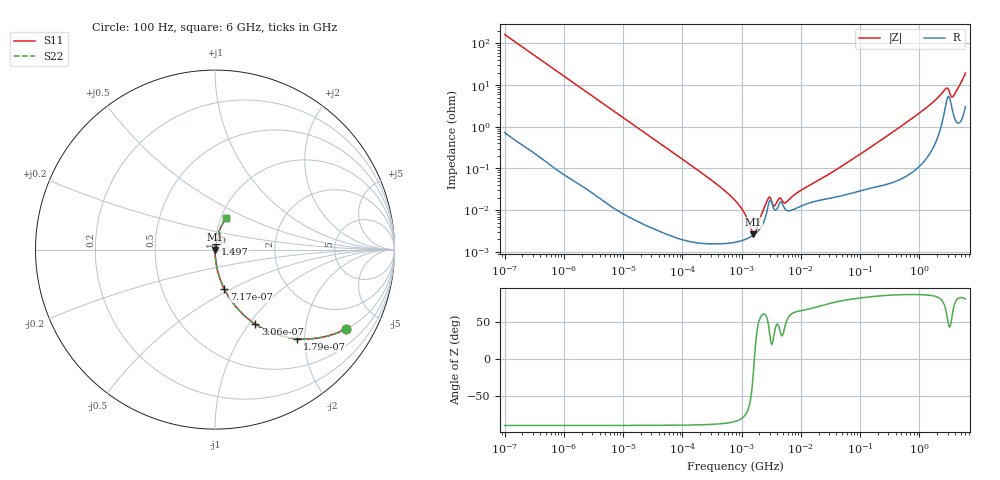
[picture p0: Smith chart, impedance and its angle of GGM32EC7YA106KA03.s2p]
!Murata Part Number: GGM32EC7YA106KA03
!These Parameters are Measured in Series Mode Connection
!Data Generated on Jun 19, 2026
!  o--ll--o
!Port1  Port2
!  o------o
!Operation Temp=25[degC], DC Bias Voltage=0[V]
!Freq. Start=100[Hz] Stop=6[GHz] 401[Steps]
# Hz S RI R 50
!Freq.(Hz) S11(Real) S11(Imag) S21(Real) S21(Imag) S12(Real) S12(Imag) S22(Real) S22(Imag)
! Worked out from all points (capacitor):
!   401 points, 100 Hz to 6 GHz, reference 50 ohm
!   read as one part in series: C = 9.68 uF near 109 Hz
!   lowest |Z| = 2.63 mohm at 1.586 MHz (marker M1)
!   series resonance near 1.645 MHz, so ESL is about 970 pH
!   S11 on the Smith chart (normalised r, x): 100 Hz: 1.01, -3.29; 179 Hz: 1.01, -1.84; 306 Hz: 1.00, -1.08; 717 Hz: 1.00, -0.46; 1.497 GHz: 1.00, +0.07; 6 GHz: 1.06, +0.38
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100  0.7288 -0.4424  0.2712 0.4424  0.2712 0.4424  0.7288 -0.4424
179  0.4582 -0.4961  0.5418 0.4961  0.5418 0.4961  0.4582 -0.4961
306  0.2255 -0.4157  0.7745 0.4157  0.7745 0.4157  0.2255 -0.4157
717  0.0512 -0.2183  0.9488 0.2183  0.9488 0.2183  0.0512 -0.2183
2008  0.00713 -0.0818  0.9929 0.0818  0.9929 0.0818  0.00713 -0.0818
40335  4.83e-05 -0.00414  1 0.00414  1 0.00414  4.83e-05 -0.00414
330837  1.57e-05 -0.000487  1 0.000487  1 0.000487  1.57e-05 -0.000487
774597  1.69e-05 -0.00017  1 0.00017  1 0.00017  1.69e-05 -0.00017
1059725  1.89e-05 -9.48e-05  1 9.48e-05  1 9.48e-05  1.89e-05 -9.48e-05
1585629  2.51e-05 -8e-06  1 8e-06  1 8e-06  2.51e-05 -8e-06
2268635  4.53e-05 7.99e-05  1 -7.99e-05  1 -7.99e-05  4.53e-05 7.99e-05
2837864  0.000133 0.000142  0.9999 -0.000142  0.9999 -0.000142  0.000133 0.000142
3549919  0.000104 7.07e-05  0.9999 -7.07e-05  0.9999 -7.07e-05  0.000104 7.07e-05
4440638  0.000153 0.000122  0.9998 -0.000122  0.9998 -0.000122  0.000153 0.000122
5554849  0.000102 0.000112  0.9999 -0.000112  0.9999 -0.000112  0.000102 0.000112
1.555665e7  0.000155 0.000396  0.9998 -0.000396  0.9998 -0.000396  0.000155 0.000396
3.124326e8  0.000475 0.00654  0.9995 -0.00654  0.9995 -0.00654  0.000475 0.00654
1.497423e9  0.00333 0.033  0.9967 -0.033  0.9967 -0.033  0.00333 0.033
2.802721e9  0.0376 0.0703  0.9624 -0.0703  0.9624 -0.0703  0.0376 0.0703
3.505958e9  0.0317 0.0391  0.9683 -0.0391  0.9683 -0.0391  0.0317 0.0391
3.8344e9  0.0206 0.0516  0.9794 -0.0516  0.9794 -0.0516  0.0206 0.0516
6e9  0.0621 0.1743  0.9379 -0.1743  0.9379 -0.1743  0.0621 0.1743
